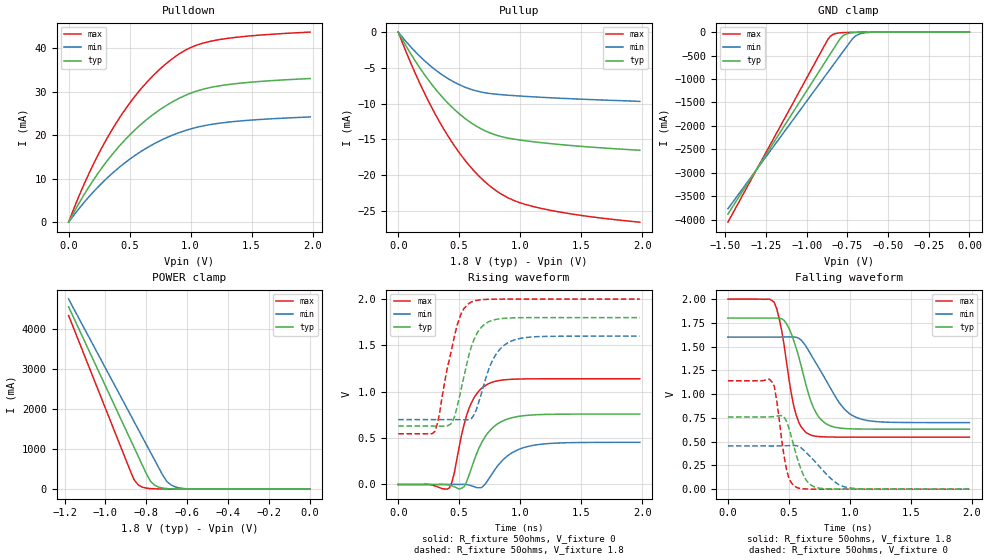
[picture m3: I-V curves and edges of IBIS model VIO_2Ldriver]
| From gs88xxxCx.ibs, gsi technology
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|  signals   DQA1-DQA9, DQB1-DQB9, DQC1-DQC9, DQD1-DQD9
[Model]   VIO_2Ldriver
Model_type   I/O
Polarity   Non-Inverting
Vinl  =   0.80v
Vinh  =   2.00v
Vmeas =   1.25v
Cref  =   0.0pF
Rref  =   50
Vref  =   1.25v
|  variable   typ   min   max
C_comp   3.0pF   2.5pF   3.5pF
|  variable   typ   min   max
[Temperature Range]   50   0   100
|  variable   typ   min   max
[Voltage Range]   1.8   1.6   2.0
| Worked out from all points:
|   slope of the pulldown table from 0 to 0.27 V, typ, clamps not added: 21.8 ohm
|   slope of the pullup table from 0 to 0.27 V, typ, clamps not added: 37.4 ohm
|   GND clamp passes 1 mA (typ) near -0.61 V on its own axis
|   POWER clamp passes 1 mA (typ) near -0.59 V on its own axis
|   rising waveform, R_fixture 50ohms, V_fixture 0: 20-80 % time 177ps typ, 207ps min, 138ps max; typ from 0 V to 0.76 V
|   rising waveform, R_fixture 50ohms, V_fixture 1.8: 20-80 % time 135ps typ, 152ps min, 134ps max; typ from 0.631 V to 1.8 V
|   falling waveform, R_fixture 50ohms, V_fixture 1.8: 20-80 % time 160ps typ, 252ps min, 113ps max; typ from 1.8 V to 0.631 V
|   falling waveform, R_fixture 50ohms, V_fixture 0: 20-80 % time 110ps typ, 204ps min, 74.9ps max; typ from 0.76 V to 0 V
[Pulldown]
| voltage   I(typ)   I(min)   I(max)
0V        -286.4pA   -891.3pA   -166.8pA
80mV      4.1mA      2.937mA    5.662mA
180mV     8.698mA    6.246mA    11.97mA
280mV     12.76mA    9.182mA    17.5mA
380mV     16.33mA    11.77mA    22.34mA
480mV     19.45mA    14.04mA    26.55mA
600mV     22.64mA    16.37mA    30.86mA
820mV     27.15mA    19.63mA    36.91mA
1V        29.64mA    21.43mA    40.13mA
1.18V     31.06mA    22.52mA    41.68mA
1.48V     32.15mA    23.43mA    42.8mA
1.98V     33.02mA    24.2mA     43.7mA
[Pullup]
| voltage (VDDQ-Vout)   I(typ)   I(min)   I(max)
0V        208.8pA    794.2pA    88.98pA
80mV      -2.401mA   -1.638mA   -3.41mA
180mV     -5.088mA   -3.433mA   -7.281mA
280mV     -7.433mA   -4.953mA   -10.73mA
380mV     -9.443mA   -6.201mA   -13.76mA
560mV     -12.24mA   -7.783mA   -18.19mA
660mV     -13.35mA   -8.306mA   -20.11mA
760mV     -14.15mA   -8.606mA   -21.64mA
920mV     -14.88mA   -8.851mA   -23.34mA
1.14V     -15.4mA    -9.086mA   -24.53mA
1.5V      -15.98mA   -9.381mA   -25.64mA
1.98V     -16.52mA   -9.69mA    -26.58mA
[GND Clamp]
| voltage   I(typ)   I(min)   I(max)
-1.485V   -3.884A    -3.771A    -4.056A
-885mV    -626.9mA   -926.9mA   -247.2mA
-870mV    -545.6mA   -856mA     -153.5mA
-855mV    -464.4mA   -785mA     -89.11mA
-825mV    -301.9mA   -643.2mA   -32.88mA
-795mV    -141.5mA   -501.4mA   -15.38mA
-780mV    -86.61mA   -430.5mA   -11.65mA
-750mV    -32.85mA   -288.8mA   -7.734mA
-705mV    -8.727mA   -95.28mA   -4.834mA
-660mV    -2.907mA   -24.97mA   -2.925mA
-555mV    -316.7uA   -1.176mA   -484.9uA
0V        -278.2pA   -874.6pA   -161.2pA
[POWER Clamp]
| voltage (VDDQ-Vout)   I(typ)   I(min)   I(max)
-1.18V    4.545A     4.74A      4.328A
-880mV    1.258A     1.875A     474.1mA
-860mV    1.039A     1.684A     234.3mA
-840mV    820.4mA    1.493A     107.4mA
-820mV    601.5mA    1.302A     50.64mA
-780mV    197.3mA    920.5mA    14.28mA
-760mV    99.71mA    729.7mA    9.034mA
-720mV    26.23mA    348.2mA    4.898mA
-700mV    13.96mA    192.6mA    3.916mA
-660mV    4.495mA    57.55mA    2.579mA
-560mV    510.5uA    2.941mA    648.3uA
0V        209pA      794.1pA    88.9pA
[Ramp]
| voltage   typ   min   max
dV/dt_r   0.92/102p   0.73/132p   1.13/79p
dV/dt_f   1.01/109p   0.86/149p   1.19/82p
R_load  =   50ohms
[Rising Waveform]
C_fixture =   0.0pF
R_fixture =   50ohms
V_fixture =   0
| Time   V(typ)   V(min)   V(max)
0s        3.884nV    15.26nV    1.766nV
420ps     -7.216mV   488.4uV    -37.09mV
460ps     -24.76mV   802.1uV    126.7mV
520ps     -39.34mV   1.143mV    540.5mV
580ps     99.61mV    -5.822mV   819.6mV
680ps     442.3mV    -34.75mV   1.034V
760ps     592.9mV    96.28mV    1.099V
880ps     698.3mV    291.7mV    1.13V
1.06ns    746.1mV    409.2mV    1.139V
1.98ns    759.6mV    454.6mV    1.14V
[Rising Waveform]
C_fixture =   0.0pF
R_fixture =   50ohms
V_fixture =   1.8
V_fixture_min =  1.6
V_fixture_max =  2.0
| Time   V(typ)   V(min)   V(max)
0s        630.9mV    699.9mV    547.1mV
300ps     630mV      699.9mV    571.5mV
340ps     629.3mV    699.8mV    778.5mV
440ps     663.4mV    700.4mV    1.472V
520ps     1.055V     698.9mV    1.857V
600ps     1.49V      711.6mV    1.969V
680ps     1.694V     974.7mV    1.993V
780ps     1.774V     1.357V     1.999V
920ps     1.796V     1.543V     2V
1.98ns    1.8V       1.6V       2V
[Falling Waveform]
C_fixture =   0.0pF
R_fixture =   50ohms
V_fixture =   1.8
V_fixture_min =  1.6
V_fixture_max =  2.0
| Time   V(typ)   V(min)   V(max)
0s        1.8V       1.6V       2V
380ps     1.8V       1.6V       1.965V
440ps     1.793V     1.601V     1.674V
540ps     1.562V     1.601V     872.6mV
640ps     1.097V     1.504V     595.6mV
700ps     859.8mV    1.373V     561.8mV
760ps     736mV      1.244V     552.1mV
920ps     642.3mV    897.1mV    547.6mV
1.04ns    633.6mV    762.5mV    547.4mV
1.98ns    631.1mV    700.2mV    547.2mV
[Falling Waveform]
C_fixture =   0.0pF
R_fixture =   50ohms
V_fixture =   0
| Time   V(typ)   V(min)   V(max)
0s        759.6mV    454.6mV    1.14V
360ps     761.5mV    454.4mV    1.13V
380ps     764.2mV    454.4mV    1.085V
400ps     768mV      454.5mV    934.7mV
480ps     715.2mV    456.9mV    208mV
560ps     362.6mV    458.1mV    20.43mV
620ps     146mV      412.4mV    3.696mV
680ps     45mV       335.6mV    813.3uV
960ps     231.6uV    22.36mV    4.995uV
1.98ns    725.2nV    1.837uV    306.5nV
